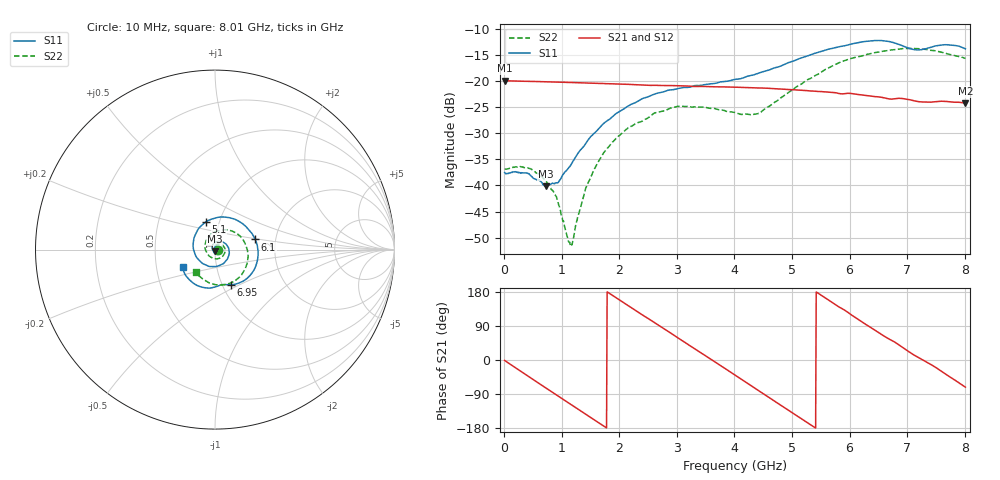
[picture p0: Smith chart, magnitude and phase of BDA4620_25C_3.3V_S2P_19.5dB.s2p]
!Agilent Technologies,E5071B,MY42404982,A.09.10
!Date: Wed May 06 08:52:54 2026
!Data & Calibration Information:
!Freq	S11:SOLT2(ON)	S21:SOLT2(ON)	S12:SOLT2(ON)	S22:SOLT2(ON)
# Hz S RI R 50
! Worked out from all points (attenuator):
!   801 points, 10 MHz to 8.01 GHz, reference 50 ohm
!   highest |S21| = -19.92 dB at 20 MHz (marker M1); lowest = -24.2 dB at 8.01 GHz (marker M2)
!   lowest |S11| = -40.2 dB at 720 MHz (marker M3), VSWR 1.02, Z = 49.9 - j0.978 ohm
!   |S11| at or under -10 dB: start of sweep to end of sweep
!   |S22| runs from -51.6 to -13.7 dB; largest |S21 - S12| = 0.00046
!   S11 on the Smith chart (normalised r, x): 10 MHz: 1.03, -0.00; 5.1 GHz: 0.86, +0.27; 6.1 GHz: 1.57, +0.19; 6.95 GHz: 1.10, -0.45; 8.01 GHz: 0.68, -0.14
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1e7  0.0133 -0.000851  0.1009 -0.00218  0.1012 -0.00217  0.0143 -0.000534
2e7  0.0131 -0.000831  0.1009 -0.00375  0.1011 -0.00413  0.0144 -0.000401
4.4e8  0.00904 -0.00912  0.0705 -0.0702  0.0705 -0.0704  0.0135 -0.00547
7.2e8  -0.000751 -0.00979  0.0285 -0.0944  0.0284 -0.0945  0.00817 -0.0077
9e8  -0.00793 -0.00707  -0.00226 -0.0979  -0.00237 -0.0982  0.00345 -0.00714
1.15e9  -0.0149 0.00409  -0.0432 -0.0869  -0.0433 -0.0871  -0.00216 -0.00148
1.19e9  -0.0155 0.00653  -0.0491 -0.0835  -0.0491 -0.0837  -0.00284 -0.000244
1.35e9  -0.0159 0.0161  -0.0698 -0.0663  -0.0699 -0.0665  -0.00456 0.00505
1.58e9  -0.0095 0.0307  -0.0893 -0.0337  -0.0894 -0.0337  -0.00385 0.0142
1.85e9  0.00818 0.0432  -0.0938 0.0101  -0.094 0.0102  0.00319 0.0246
2.16e9  0.0369 0.0447  -0.0743 0.0561  -0.0744 0.0562  0.0183 0.0306
2.68e9  0.0768 0.00507  -0.00312 0.0909  -0.00296 0.091  0.0463 0.0196
3.08e9  0.071 -0.0489  0.0549 0.0714  0.0552 0.0714  0.0568 -0.00878
4.01e9  -0.0699 -0.0767  0.0672 -0.056  0.0673 -0.0561  -0.0125 -0.0484
4.42e9  -0.1192 -0.0017  0.0139 -0.0847  0.0139 -0.0847  -0.0476 -0.0128
5.1e9  -0.0519 0.1534  -0.0702 -0.0426  -0.0704 -0.0425  -0.0193 0.0878
5.35e9  0.0188 0.1802  -0.0798 -0.00891  -0.0799 -0.00889  0.0237 0.1056
6.1e9  0.2244 0.0564  -0.028 0.0697  -0.0281 0.0699  0.1638 0.0421
6.68e9  0.1773 -0.1617  0.038 0.0558  0.0382 0.0559  0.173 -0.0948
6.95e9  0.089 -0.1953  0.0588 0.0336  0.0589 0.0336  0.1352 -0.1542
7.58e9  -0.0684 -0.2102  0.0565 -0.0304  0.0566 -0.0304  -0.0233 -0.1887
8.01e9  -0.1804 -0.0952  0.0193 -0.0583  0.0195 -0.0584  -0.1067 -0.1256
